DATA_BLOCK "ALLARMI_MP270"
AUTHOR : LD
FAMILY : DESTACK
NAME : ALLARMI
VERSION : 0.1


  STRUCT
   Allar_9 : BOOL ;	//Magnetotermici 24 Volt drive
   Allar_10 : BOOL ;	//Magnetotermico alimentazione uscite plc
   Allar_11 : BOOL ;	//Magnetotermico alimentazione ingressi plc
   Allar_12 : BOOL ;	//Magnetotermico traslazione tavola 1
   Allar_13 : BOOL ;	//Magnetotermico traslazione tavola 2
   Allar_14 : BOOL ;	//Magnetotermico pompa tavola 1
   Allar_15 : BOOL ;	//Magnetotermico pompa tavola 2
   Allar_16 : BOOL ;	//Magnetotermico regolazione altezza sfogliatore
   Allar_1 : BOOL ;	//Emergenze da ripristinare
   Allar_2 : BOOL ;	//Emergenza pannello di comando
   Allar_3 : BOOL ;	//Emergenza sfogliatore lato operatore
   Allar_4 : BOOL ;	//Emergenza porta sfogliatore lato opposto operatore
   Allar_5 : BOOL ;	//Emergenza porta lato operatore
   Allar_6 : BOOL ;	//Emergenza porta lato opposto operatore
   Allar_7 : BOOL ;	//Porta aperta lato operatore
   Allar_8 : BOOL ;	//Porta aperta lato opposto operatore
   Allar_25 : BOOL ;	//Magnetotermico ventilatore armadio
   Allar_26 : BOOL ;	//Magnetotermico generale ausiliari
   Allar_27 : BOOL ;	//Antischiacciamento tavola 1 sx
   Allar_28 : BOOL ;	//Antischiacciamento tavola 2 dx
   Allar_29 : BOOL ;	//Anticollisione tavola 1 sx
   Allar_30 : BOOL ;	//Anticollisione tavola 2 dx
   Allar_31 : BOOL ;	//Oltrecorsa salita tavola
   Allar_32 : BOOL ;	//Barriera di sicurezza dx lato opposto operatore
   Allar_17 : BOOL ;	//Magnetotermico regolazione altezza centratore
   Allar_18 : BOOL ;	//Magnetotermico traslazione centratore
   Allar_19 : BOOL ;	//Magnetotermico regolazione posteriore sx centratore
   Allar_20 : BOOL ;	//Magnetotermico regolazione posteriore dx centratore
   Allar_21 : BOOL ;	//Magnetotermico regolazione anteriore sx centratore
   Allar_22 : BOOL ;	//Magnetotermico regolazione anteriore dx centratore
   Allar_23 : BOOL ;	//Magnetotermico regolazione laterale dx centratore
   Allar_24 : BOOL ;	//Magnetotermico regolazione laterale sx centratore
   Allar_41 : BOOL ;	//Sicurezze antischiacc.e anticollisione escluse
   Allar_42 : BOOL ;	//Disfunzione micro P.E. su centratore
   Allar_43 : BOOL ;	//Riserva
   Allar_44 : BOOL ;	//Selezione cambio produzione manuale inserito
   Allar_45 : BOOL ;	//Richiesta apertura isola 1
   Allar_46 : BOOL ;	//Anomalia drive centratore Posteriore DX
   Allar_47 : BOOL ;	//Anomalia drive centratore Laerale DX
   Allar_48 : BOOL ;	//Anomalia drive centratore Laerale SX
   Allar_33 : BOOL ;	//Allarme su AP&T
   Allar_34 : BOOL ;	//Matricola non caricata da AP&T
   Allar_35 : BOOL ;	//Magneti non in posizione
   Allar_36 : BOOL ;	//Portare AP&T in posizione di inizio ciclo
   Allar_37 : BOOL ;	//Anomalia drive centratore Anteriore DX
   Allar_38 : BOOL ;	//Anomalia drive centratore Anteriore SX
   Allar_39 : BOOL ;	//Anomalia drive centratore Posteriore DX
   Allar_40 : BOOL ;	//Posizionare ABB in cambio produzione
   Allar_57 : BOOL ;	//Fine pacco tranciati su tavola
   Allar_58 : BOOL ;	//Riserva
   Allar_59 : BOOL ;	//Pressa non al P.M.S.
   Allar_60 : BOOL ;	//Spina start pressa non inserita
   Allar_61 : BOOL ;	//FC TAVOLA 1 lato disimpilamento
   Allar_62 : BOOL ;	//FC TAVOLA 2 lato disimpilamento
   Allar_63 : BOOL ;	//Allarme da robot perdita pezzo
   Allar_64 : BOOL ;	//Allarme riparo aperto isola 1
   Allar_49 : BOOL ;	//Lamiera nello stampo
   Allar_50 : BOOL ;	//Lamiera su centraggio in ciclo di cambio produzione
   Allar_51 : BOOL ;	//Pressa non pronta per auto
   Allar_52 : BOOL ;	//Doppio foglio
   Allar_53 : BOOL ;	//Robot non pronto per auto
   Allar_54 : BOOL ;	//Assenza foglio su stazione di centraggio
   Allar_55 : BOOL ;	//Braccio ABB non in posizione di produzione
   Allar_56 : BOOL ;	//Attesa pezzo prelevato dallo stampo (robot isola1)
   Allar_73 : BOOL ;	//Ciclo cambio matricola in corso
   Allar_74 : BOOL ;	//Ciclo cambio pacco in corso
   Allar_75 : BOOL ;	//Sicurezza magneti sfogliatore
   Allar_76 : BOOL ;	//Pacco non arrivato in posizione di sfogliatura
   Allar_77 : BOOL ;	//Tavola 1 non in finecorsa lato caricamento (indietro
   Allar_78 : BOOL ;	//Tavola 2 non in finecorsa lato caricamento (indietro
   Allar_79 : BOOL ;	//Magneti sfogliatori non rientrati
   Allar_80 : BOOL ;	//Riserva
   Allar_65 : BOOL ;	//Barriera di sicurezza sx lato operatore
   Allar_66 : BOOL ;	//cancelletti tavola 1
   Allar_67 : BOOL ;	//cancelletti tavola 2x
   Allar_68 : BOOL ;	//Unita' di centraggio sbloccata
   Allar_69 : BOOL ;	//Cambio matricola quota non raggiunta
   Allar_70 : BOOL ;	//Batteria plc scarica
   Allar_71 : BOOL ;	//Tavola 1 non abbassata
   Allar_72 : BOOL ;	//Tavola 2 non abbassata
   Allar_89 : BOOL ;	//Contemporaneita' fc  traslazione tavola 1
   Allar_90 : BOOL ;	//Contemporaneita' fc  traslazione tavola 2
   Allar_91 : BOOL ;	//Contemporaneita' fc regolazione altezza sfogliatore
   Allar_92 : BOOL ;	//Contemporaneita' fc  regolazione altezza centraggio
   Allar_93 : BOOL ;	//Contemporaneita' fc  traslazione centratore
   Allar_94 : BOOL ;	//Contemporaneita' fc  regolazione centraggio post.SX
   Allar_95 : BOOL ;	//Contemporaneita' fc  regolazione centraggio post.DX
   Allar_96 : BOOL ;	//Contemporaneita' fc  regolazione centraggio ant.
   Allar_81 : BOOL ;	//Muting inserito tavola 1
   Allar_82 : BOOL ;	//Muting inserito tavola 2
   Allar_83 : BOOL ;	//Comandi disinseriti
   Allar_84 : BOOL ;	//Braccio ABB in posizione di prelievo
   Allar_85 : BOOL ;	//Anomalia vuoto su centratore
   Allar_86 : BOOL ;	//Anomalia vuoto su sfogliatore
   Allar_87 : BOOL ;	//Quota tavola non raggiunta
   Allar_88 : BOOL ;	//Selettore programmazione inserito
   Allar_105 : BOOL ;	//Anomalia fc  tavola 1 avanti lato dispilamento
   Allar_106 : BOOL ;	//Anomalia fc  tavola 1 indietro lato carico
   Allar_107 : BOOL ;	//Anomalia fc  tavola 2 avanti lato dispilamento
   Allar_108 : BOOL ;	//Anomalia fc  tavola 2 indietro lato carico
   Allar_109 : BOOL ;	//Zero assi centratore da eseguire
   Allar_110 : BOOL ;	//Inserire nuovo codice matricola
   Allar_111 : BOOL ;	//Sostituire tooling e premere C.P. start
   Allar_112 : BOOL ;	//Tavola di centraggio non bloccata
   Allar_97 : BOOL ;	//Selezione cambio produzione in automatico
   Allar_98 : BOOL ;	//Contemporaneita' fc  centratura laterale dx
   Allar_99 : BOOL ;	//Contemporaneita' fc centratura laterale sx
   Allar_100 : BOOL ;	//Time out centraggi longitudinali fuori
   Allar_101 : BOOL ;	//Time out centraggi laterale fuori
   Allar_102 : BOOL ;	//Contemporaneita' fc blocc/sblocc centratore
   Allar_103 : BOOL ;	//Contemporaneita' fc  sollevamento tavola 1
   Allar_104 : BOOL ;	//Contemporaneita' fc  sollevamento tavola 2
   Allar_121 : BOOL ;	//Assenza pedana materiale su tavola zona sfogliatura
   Allar_122 : BOOL ;	//Fotocellula 45B1 H200 guasta o disallineata
   Allar_123 : BOOL ;	//Fotocellula 45B3 H120 guasta o disallineata
   Allar_124 : BOOL ;	//Salire con la tavola in manuale
   Allar_125 : BOOL ;	//Anomalia dispositivo Klaska (cavo interrotto)
   Allar_126 : BOOL ;	//Time out Unita' di centraggio bloccata
   Allar_127 : BOOL ;	//Time out Unita' di centraggio sbloccata
   Allar_128 : BOOL ;	//Magnetotermico trasformatore brushless centratori (12QF2)
   Allar_113 : BOOL ;	//Motori ABB non inseriti
   Allar_114 : BOOL ;	//Cambio pacco prenotato
   Allar_115 : BOOL ;
   Allar_116 : BOOL ;	//Tavole 1 e 2  in muting
   Allar_117 : BOOL ;	//Klascka non rileva sequenza 2Fogli, 1Foglio, 0Fogli
   Allar_118 : BOOL ;	//Klascka non rileva 2 fogli nel prelievo
   Allar_119 : BOOL ;	//Klascka rileva 0 fogli nel ciclo di carico
   Allar_120 : BOOL ;	//Braccio ABB non in posizione di prelievo
   Allar_137 : BOOL ;	//Time out salita regolazione altezza centratore
   Allar_138 : BOOL ;	//Time out discesa regolazione altezza centratore
   Allar_139 : BOOL ;	//Time out centratore verso pressa
   Allar_140 : BOOL ;	//Time out centratore verso sfogliatore
   Allar_141 : BOOL ;	//Time out indietro magnete 1
   Allar_142 : BOOL ;	//Time out avanti magnete 1
   Allar_143 : BOOL ;	//Time out indietro magnete 2
   Allar_144 : BOOL ;	//Time out avanti magnete 2
   Allar_129 : BOOL ;	//Contemporaneita' fc magnete 1
   Allar_130 : BOOL ;	//Contemporaneita' fc magnete 2
   Allar_131 : BOOL ;	//Contemporaneita' fc magnete 3
   Allar_132 : BOOL ;	//Contemporaneita' fc magnete 4
   Allar_133 : BOOL ;	//Contemporaneita' fc magnete 5
   Allar_134 : BOOL ;	//Contemporaneita' fc magnete 6
   Allar_135 : BOOL ;	//Contemporaneita' fc magnete laterale sx
   Allar_136 : BOOL ;	//Contemporaneita' fc magnete laterale dx
   Allar_153 : BOOL ;	//Time out indietro magnete laterale sx
   Allar_154 : BOOL ;	//Time out avanti magnete laterale sx
   Allar_155 : BOOL ;	//Time out indietro magnete laterale dx
   Allar_156 : BOOL ;	//Time out avanti magnete laterale dx
   Allar_157 : BOOL ;	//Time out chiusura braccio magnete laterale sx
   Allar_158 : BOOL ;	//Time out apertura braccio magnete laterale sx
   Allar_159 : BOOL ;	//Time out chiusura braccio magnete laterale dx
   Allar_160 : BOOL ;	//Time out apertura braccio magnete laterale dx
   Allar_145 : BOOL ;	//Time out indietro magnete 3
   Allar_146 : BOOL ;	//Time out avanti magnete 3
   Allar_147 : BOOL ;	//Time out indietro magnete 4
   Allar_148 : BOOL ;	//Time out avanti magnete 4
   Allar_149 : BOOL ;	//Time out indietro magnete 5
   Allar_150 : BOOL ;	//Time out avanti magnete 5
   Allar_151 : BOOL ;	//Time out indietro magnete 6
   Allar_152 : BOOL ;	//Time out avanti magnete 6
   Allar_169 : BOOL ;	//Porta aperta sfogliatore lato dx
   Allar_170 : BOOL ;	//Porta aperta sfogliatore lato sx
   Allar_171 : BOOL ;	//Extracorsa avanti tavola 1
   Allar_172 : BOOL ;	//Extracorsa avanti tavola 2
   Allar_173 : BOOL ;	//Extracorsa indietro tavola 1
   Allar_174 : BOOL ;	//Extracorsa indietro tavola 2
   Allar_175 : BOOL ;	//Emergenza ABB
   Allar_176 : BOOL ;	//Extracorsa incremento pacco (fc su braccio ABB)
   Allar_161 : BOOL ;	//Carro non in posizione di riposo
   Allar_162 : BOOL ;	//Periferia decentrata Destacker in errore
   Allar_163 : BOOL ;	//Periferia decentrata AP&T in errore
   Allar_164 : BOOL ;	//Ciclo AP&T non coerente
   Allar_165 : BOOL ;	//E60.4 Magnete Ausiliario 1 Tavola 1 non rientrato
   Allar_166 : BOOL ;	//E60.6 Magnete Ausiliario 2 Tavola 1 non rientrato
   Allar_167 : BOOL ;	//E70.4 Magnete Ausiliario 1 Tavola 2 non rientrato
   Allar_168 : BOOL ;	//E70.6 Magnete Ausiliario 2 Tavola 2 non rientrato
   Allar_185 : BOOL ;	//Attenzione!  dovresti aprire i centraggi
   Allar_186 : BOOL ;	//Emergenza linea Comau da ripristinare
   Allar_187 : BOOL ;	//Ripristinare sensore presenza su braccio ABB
   Allar_188 : BOOL ;	//Mancanza improvvisa consenso ingr.pressa
   Allar_189 : BOOL ;	//ABB non in start auto  (ciclo in corso)
   Allar_190 : BOOL ;	//Posizionare i gruppi a riposo per cambio tooling
   Allar_191 : BOOL ;	//Retrofitting pulsanti EM non premuti per comau
   Allar_192 : BOOL ;	//Retrofitting Ripari chiusi per ABB
   Allar_177 : BOOL ;	//Tavola 1 piena in uscita
   Allar_178 : BOOL ;	//Tavola 2 piena in uscita
   Allar_179 : BOOL ;	//Retrofitting rele' ciclo automatico destacker
   Allar_180 : BOOL ;	//Retrofitting rele' ripari/barriere destacker
   Allar_181 : BOOL ;	//Retrofitting rele' start pressa (per comau)
   Allar_182 : BOOL ;	//Retrofitting Rele' emergenza Destaker
   Allar_183 : BOOL ;	//Retrofitting anticollisione/antischiacciamento tavole
   Allar_184 : BOOL ;	//Retrofitting override barriere
   word_3042 : BOOL ;
   word_3043 : BOOL ;
   word_3044 : BOOL ;
   word_3045 : BOOL ;
   word_3046 : BOOL ;
   word_3047 : BOOL ;
   word_3048 : BOOL ;
   word_3049 : BOOL ;
   word_3050 : BOOL ;
   word_3051 : BOOL ;
   word_3052 : BOOL ;
   word_3053 : BOOL ;
   word_3054 : BOOL ;
   word_3055 : BOOL ;
   word_3056 : BOOL ;
   word_3057 : BOOL ;
   Allar_217 : BOOL ;	//Porta 2: non abilitata alla marcia
   Allar_218 : BOOL ;	//Porta 2: time-out discesa porta o non chiusa
   Allar_219 : BOOL ;	//Porta 2: time-out salita porta o non aperta
   Allar_220 : BOOL ;	//Porta 2: carro non in posizione per ciclo porta
   Allar_221 : BOOL ;	//Porta 2: livello di traslazione carro 2 troppo alto
   word_3063 : BOOL ;
   word_3064 : BOOL ;
   word_3065 : BOOL ;
   Allar_209 : BOOL ;	//Porta 1: non abilitata alla marcia
   Allar_210 : BOOL ;	//Porta 1: time-out discesa porta o non chiusa
   Allar_211 : BOOL ;	//Porta 1: time-out salita porta o non aperta
   Allar_212 : BOOL ;	//Porta 1: carro non in posizione per ciclo porta
   Allar_213 : BOOL ;	//Porta 1: livello di traslazione carro 1 troppo alto
   word_30635 : BOOL ;
   word_30636 : BOOL ;
   word_30637 : BOOL ;
   word_30638 : BOOL ;
   word_30639 : BOOL ;
   word_306310 : BOOL ;
   word_306311 : BOOL ;
   word_306312 : BOOL ;
   word_306313 : BOOL ;
   word_306314 : BOOL ;
   word_306315 : BOOL ;
   Allar_225 : BOOL ;	//Porta 1 e 2: magnetotermico linea alimentazione porte 1 e 2
   word_3063152 : BOOL ;
   word_3063153 : BOOL ;
   word_30631531 : BOOL ;
   word_30631532 : BOOL ;
   word_30631533 : BOOL ;
   word_30631534 : BOOL ;
   word_30631535 : BOOL ;
   Da_APT_allarme_1 : BOOL ;	//SF1 - A: Pezzo caduto in pinza I @1D%5.1f@
   Da_APT_allarme_2 : BOOL ;	//SF1 - M: Non riceve il pezzo nella pinza I@1D%5.1f@
   Da_APT_allarme_3 : BOOL ;	//SF1 - W: Intermittenza vuoto troppo elevata nell'unità di presa I@1D%5.1f@
   Da_APT_allarme_4 : BOOL ;	//SF1 - A: Errore unità di presa protezione vuoto I@1D%5.1f@
   Da_APT_allarme_5 : BOOL ;	//SF1 - W: Errore unità di presa aperta I@1D%5.1f@
   Da_APT_allarme_6 : BOOL ;	//SF1 - A: Comando stop salto sequenza
   Da_APT_allarme_7 : BOOL ;	//SF1 - M: Avvio forzato
   Da_APT_allarme_8 : BOOL ;	//SF1 - A: L'asse X1_A1 ha perduto la regolazione
   Da_APT_allarme_9 : BOOL ;	//SF1 - A: Doppio Foglio UC70
   Da_APT_allarme_10 : BOOL ;	//SF1 – A: Errore di calibrazione controllo Doppio Foglio UC70
   Da_APT_allarme_11 : BOOL ;	//SF1 - M: Assi non innestati
   Da_APT_allarme_12 : BOOL ;	//SF1 - A: Perdita innesto assi
   Da_APT_allarme_13 : BOOL ;	//RISERVA
   Da_APT_allarme_14 : BOOL ;	//SF1 - A: Posizione o salto fuori limiti - fase - Check MP177
   Da_APT_allarme_15 : BOOL ;	//SF1 - A: Errore coordinate parametri di impilamento 1
   Da_APT_allarme_16 : BOOL ;	//SF1 - A: Timeout per richiesta apertura protezione
   Da_APT_allarme_17 : BOOL ;	//SF1 - A: Errore avanzamento asse
   Da_APT_allarme_18 : BOOL ;	//SF1 - A: Errore calibrazione asse
   Da_APT_allarme_19 : BOOL ;	//SF1 - M: Movimento in Z- non possibile per intervento Klaschka
   Da_APT_allarme_20 : BOOL ;	//SF1 - A: Timeout per misurazione/calibrazione nel controllo Doppio Foglio
   Da_APT_allarme_21 : BOOL ;	//SF1 - M: Quantità impostata raggiunta - contatore 1
   Da_APT_allarme_22 : BOOL ;	//SF1 - M: Quantità impostata raggiunta - contatore 2
   Da_APT_allarme_23 : BOOL ;	//SF1 - A: Stop da Linea
   Da_APT_allarme_24 : BOOL ;	//RISERVA
   Da_APT_allarme_25 : BOOL ;	//SF1 - A: Ripari aperti
   Da_APT_allarme_26 : BOOL ;	//A1624 – M:Intervento disgiuntore, controllare alimentazione a unità QF860
   Da_APT_allarme_27 : BOOL ;	//SF1  A: Nessun dettaglio trovato sulla navetta di alimentazione
   Da_APT_allarme_28 : BOOL ;	//SF1 - A: Parte imprevista su navetta
   Da_APT_allarme_29 : BOOL ;	//SF1 - M: Ripari aperti o non ripristinati
   Da_APT_allarme_30 : BOOL ;	//RISERVA
   Da_APT_allarme_31 : BOOL ;	//RISERVA
   Da_APT_allarme_32 : BOOL ;	//RISERVA
   Da_APT_allarme_33 : BOOL ;	//RISERVA
   Da_APT_allarme_34 : BOOL ;	//SF1 - M: Timeout cambio ricetta
   Da_APT_allarme_35 : BOOL ;	//A1624 - M: Trasportatore pieno
   Da_APT_allarme_36 : BOOL ;	//A1624 - A: Interruttore del nastro trasportatore scattato
   Da_APT_allarme_37 : BOOL ;	//A1624 - M:Arresto di emergenza interno attivato
   Da_APT_allarme_38 : BOOL ;	//SF1 - M: Pallet 1 completo - Cambiare pallet
   Da_APT_allarme_39 : BOOL ;	//SF1 - M: Pallet 2 completo - Cambiare pallet
   Da_APT_allarme_40 : BOOL ;	//SF1 - A: Arresto da controllo estrattore
   Da_APT_allarme_41 : BOOL ;	//SF1 - M: Nessuna parte in posizione su navetta
   Da_APT_allarme_42 : BOOL ;	//SF1 - A: Parte imprevista su navetta
   Da_APT_allarme_43 : BOOL ;	//SF1 - A: L'asse X1_A1 ha perduto la regolazione
   Da_APT_allarme_44 : BOOL ;	//SF1 - A: L'asse Y_A1 ha perduto la regolazione
   Da_APT_allarme_45 : BOOL ;	//SF1 - A: L'asse Z_A1 ha perduto la regolazione
   Da_APT_allarme_46 : BOOL ;	//SF1 - A: L'asse A_A1 ha perduto la regolazione
   Da_APT_allarme_47 : BOOL ;	//SF1 - A: Pressa non in posizione superiore
   Da_APT_allarme_48 : BOOL ;	//SF1 - A: Basculamento non alto
   Da_APT_allarme_49 : BOOL ;	//A1624 - W: Guasto nella navetta del motore dell'attacco laterale
   Da_APT_allarme_50 : BOOL ;	//A1624 - A: Nessuna connessione al PLC A500 di sicurezza
   Da_APT_allarme_51 : BOOL ;	//RISERVA
   Da_APT_allarme_52 : BOOL ;	//SF1 - A: Errore di sicurezza integrata. Ripristinare la SI o riavviare
   Da_APT_allarme_53 : BOOL ;	//SF1 - A: Parte rilasciata, unità di presa troppo calda
   Da_APT_allarme_54 : BOOL ;	//SF1 - A: Timeout per unità di presa calda, azionare per sfridi
   Da_APT_allarme_55 : BOOL ;	//SF1 - M:Timeout per unità di presa calda, lasciare parte nell'utensile
   Da_APT_allarme_56 : BOOL ;	//SF1 - W: Protezione da surriscaldamento per pinza bloccata
   Da_APT_allarme_57 : BOOL ;	//SF1 A: il valore limite pressa non rientra nell'intervallo programmato
   Da_APT_allarme_58 : BOOL ;	//A1624 - g_i_ERROR[58]
   Da_APT_allarme_59 : BOOL ;	//A1624 - g_i_ERROR[59]
   Da_APT_allarme_60 : BOOL ;	//A1624 - g_i_ERROR[60]
   Da_APT_allarme_61 : BOOL ;	//A1624 - g_i_ERROR[61]
   Da_APT_allarme_62 : BOOL ;	//RISERVA
   Da_APT_allarme_63 : BOOL ;	//RISERVA
   Da_APT_allarme_64 : BOOL ;	//RISERVA
   Da_APT_allarme_65 : BOOL ;	//RISERVA
   Da_APT_allarme_66 : BOOL ;	//RISERVA
   Da_APT_allarme_67 : BOOL ;	//RISERVA
   Da_APT_allarme_68 : BOOL ;	//RISERVA
   Da_APT_allarme_69 : BOOL ;	//RISERVA
   Da_APT_allarme_70 : BOOL ;	//A1624 - M: Nessuna comunicazione - unità linea
   Da_APT_allarme_71 : BOOL ;	//A1624 - W: Tensione batteria bassa K600
   Da_APT_allarme_72 : BOOL ;	//A1624 - A: Errore dell'unità servoalimentatore TA700 - UH1
   Da_APT_allarme_73 : BOOL ;	//A1624 - A: Malfunzionamento nel contattore principale QA700 -UH1
   Da_APT_allarme_74 : BOOL ;	//RISERVA
   Da_APT_allarme_75 : BOOL ;	//A1624 - M: Modalità test attiva
   Da_APT_allarme_76 : BOOL ;	//SF1 - A: Arresto di emergenza interno MP177. K75-1
   Da_APT_allarme_77 : BOOL ;	//A1624 - A: Arresto di emergenza esterno
   Da_APT_allarme_78 : BOOL ;	//A1624 - A: Feedback safe 24V non OK - S
   Da_APT_allarme_79 : BOOL ;	//SF1 - A: Sovraccarico asse X1_A1
   Da_APT_allarme_80 : BOOL ;	//SF1 - A: Sovraccarico asse Z_A1
   Da_APT_allarme_81 : BOOL ;	//SF1 - A: Sovraccarico asse Y_A1
   Da_APT_allarme_82 : BOOL ;	//SF1 - A: Sovraccarico asse A_A1
   Da_APT_allarme_83 : BOOL ;	//A1624 - M: Livello dell'olio dell'unità di lubrificazione basso
   Da_APT_allarme_84 : BOOL ;	//A1624 - g_i_ERROR[84]
   Da_APT_allarme_85 : BOOL ;	//A1624 - g_i_ERROR[85]
   Da_APT_allarme_86 : BOOL ;	//A1624 - g_i_ERROR[86]
   Da_APT_allarme_87 : BOOL ;	//A1624 - g_i_ERROR[87]
   Da_APT_allarme_88 : BOOL ;	//RISERVA
   Da_APT_allarme_89 : BOOL ;	// - M: Unità di lubrificazione non accesa
   Da_APT_allarme_90 : BOOL ;	//A1624 - A: Il cilindro raccoglitore HSD non riceve il vuoto
   Da_APT_allarme_91 : BOOL ;	//A1624 - M: Raspa non in pos. interna HSD
   Da_APT_allarme_92 : BOOL ;	//A1624 - A: Telaio di sicurezza HSD scattato
   Da_APT_allarme_93 : BOOL ;	//A1624 - A: Deposito HSD non in posizione
   Da_APT_allarme_94 : BOOL ;	//SF1 - A: Assi esterni ai limiti dell'accoppiamento automatico
   Da_APT_allarme_95 : BOOL ;	//SF1 - M: Parametri di manovra modificati - Riavviare controllo sistema
   Da_APT_allarme_96 : BOOL ;	//SF1 - A: Errore di download dei parametri
   Da_APT_allarme_97 : BOOL ;	//BF - M: Protezioni aperte o non ripristinate - Deposito 1
   Da_APT_allarme_98 : BOOL ;	//BF - M: Protezioni aperte o non ripristinate - Deposito 2
   Da_APT_allarme_99 : BOOL ;	//A1624 - M: Ripristino della sicurezza integrata
   Da_APT_allarme_100 : BOOL ;	//A1624 - M: Fusibile F1 scattato - Armadio UH1
   Da_APT_allarme_101 : BOOL ;	//A1624 - M: Fusibile F5 scattato - Armadio UH1
   Da_APT_allarme_102 : BOOL ;	//A1624 - M: Fusibile F6 scattato - Armadio UH1
   Da_APT_allarme_103 : BOOL ;	//A1624 - M: Fusibile F860 scattato - Armadio UH1
   Da_APT_allarme_104 : BOOL ;	//A1624 - W: Unità di raffreddamento non funzionante - Armadio UH1
   Da_APT_allarme_105 : BOOL ;	//A1624 - A: Profisafe I/O richiede conferma
   Da_APT_allarme_106 : BOOL ;	//A1624 - A: Feedback per arresto di emergenza non OK I17.0
   Da_APT_allarme_107 : BOOL ;	//A1624 - A: Arresto di emergenza interno ARxxx
   Da_APT_allarme_108 : BOOL ;	//A1624 - A: Arresto di emergenza interno ARxxx
   Da_APT_allarme_109 : BOOL ;	//A1624 - A: Arresto di emergenza interno MP177 COIL
   Da_APT_allarme_110 : BOOL ;	//A1624 - M: Fusibile F1 scattato - Armadio UH2
   Da_APT_allarme_111 : BOOL ;	//A1624 - M: Fusibile F5 scattato - Armadio UH2
   Da_APT_allarme_112 : BOOL ;	//A1624 - M: Fusibile F6 scattato - Armadio UH2
   Da_APT_allarme_113 : BOOL ;	//A1624 - M: Fusibile F860 scattato - Armadio UH2
   Da_APT_allarme_114 : BOOL ;	//A1624 - W: Unità di raffreddamento non operativo - Cabinet UH2
   Da_APT_allarme_115 : BOOL ;	//SF1 - A: Errore dell'asse X1_A1
   Da_APT_allarme_116 : BOOL ;	//SF1 - A: Errore dell'asse Z_A1
   Da_APT_allarme_117 : BOOL ;	//SF1 - A: Errore dell'asse Y_A1
   Da_APT_allarme_118 : BOOL ;	//SF1 - A: Errore dell'asse A_A1
   Da_APT_allarme_119 : BOOL ;	//RISERVA
   Da_APT_allarme_120 : BOOL ;	//SF1 - A: Arresto dalla macchina esterna - PS1 (Pressa)
   Da_APT_allarme_121 : BOOL ;	//SF1 - A: Arresto dalla macchina esterna - PS2 (Comau robot)
   Da_APT_allarme_122 : BOOL ;	//SF1 - A: Arresto dalla macchina esterna - PS3
   Da_APT_allarme_123 : BOOL ;	//SF1 - A: Arresto dalla macchina esterna - PS4
   Da_APT_allarme_124 : BOOL ;	//SF1 - A: Perdita pezzo - Sfogliatore - I10.4
   Da_APT_allarme_125 : BOOL ;	//SF1 - A: Perdita pezzo - Sfogliatore - I10.5
   Da_APT_allarme_126 : BOOL ;	//SF1 - A: Perdita pezzo - Centraggio - I10.6
   Da_APT_allarme_127 : BOOL ;	//SF1 - A: Perdita pezzo - Centraggio - I10.7
   Da_APT_allarme_128 : BOOL ;	//SF1 - M: Pezzo non prelevato - Sfogliatore - I10.4
   Da_APT_allarme_129 : BOOL ;	//SF1 - M: Pezzo non prelevato - Sfogliatore - I10.5
   Da_APT_allarme_130 : BOOL ;	//SF1 - M: Pezzo non prelevato - Centraggio - I10.6
   Da_APT_allarme_131 : BOOL ;	//SF1 - M: Pezzo non prelevato - Centraggio - I10.7
   Da_APT_allarme_132 : BOOL ;	//SF1 - W: Amolalia vuoto - Sfogliatore - I10.4
   Da_APT_allarme_133 : BOOL ;	//SF1 - W: Amolalia vuoto - Sfogliatore - I10.5
   Da_APT_allarme_134 : BOOL ;	//SF1 - W: Amolalia vuoto - Centraggio - I10.6
   Da_APT_allarme_135 : BOOL ;	//SF1 - W: Amolalia vuoto - Centraggio - I10.7
   Da_APT_allarme_136 : BOOL ;	//SF1 - A: Anomalia vacuostato - Sfogliatore - I10.4
   Da_APT_allarme_137 : BOOL ;	//SF1 - A: Anomalia vacuostato - Sfogliatore - I10.5
   Da_APT_allarme_138 : BOOL ;	//SF1 - A: Anomalia vacuostato - Centraggio - I10.6
   Da_APT_allarme_139 : BOOL ;	//SF1 - A: Anomalia vacuostato - Centraggio - I10.7
   Da_APT_allarme_140 : BOOL ;	//SF1 - M: Richiesta Svuotamento Linea
   Da_APT_allarme_141 : BOOL ;	//SF1 - A: Spare application Nr 10
   Da_APT_allarme_142 : BOOL ;	//SF1 - A: Spare application Nr 9
   Da_APT_allarme_143 : BOOL ;	//SF1 - A: Spare application Nr 8
   Da_APT_allarme_144 : BOOL ;	//SF1 - A: Spare application Nr 7
   Da_APT_allarme_145 : BOOL ;
   Da_APT_allarme_146 : BOOL ;
   Da_APT_allarme_147 : BOOL ;
   Da_APT_allarme_148 : BOOL ;
   Da_APT_allarme_149 : BOOL ;
   Da_APT_allarme_150 : BOOL ;
   Da_APT_allarme_151 : BOOL ;
   Da_APT_allarme_152 : BOOL ;
   Da_APT_allarme_153 : BOOL ;
   Da_APT_allarme_154 : BOOL ;
   Da_APT_allarme_155 : BOOL ;
   Da_APT_allarme_156 : BOOL ;
   Da_APT_allarme_157 : BOOL ;
   Da_APT_allarme_158 : BOOL ;
   Da_APT_allarme_159 : BOOL ;
   Da_APT_allarme_160 : BOOL ;
  END_STRUCT ;
BEGIN
   Allar_9 := FALSE;
   Allar_10 := FALSE;
   Allar_11 := FALSE;
   Allar_12 := FALSE;
   Allar_13 := FALSE;
   Allar_14 := FALSE;
   Allar_15 := FALSE;
   Allar_16 := FALSE;
   Allar_1 := FALSE;
   Allar_2 := FALSE;
   Allar_3 := FALSE;
   Allar_4 := FALSE;
   Allar_5 := FALSE;
   Allar_6 := FALSE;
   Allar_7 := FALSE;
   Allar_8 := FALSE;
   Allar_25 := FALSE;
   Allar_26 := FALSE;
   Allar_27 := FALSE;
   Allar_28 := FALSE;
   Allar_29 := FALSE;
   Allar_30 := FALSE;
   Allar_31 := FALSE;
   Allar_32 := FALSE;
   Allar_17 := FALSE;
   Allar_18 := FALSE;
   Allar_19 := FALSE;
   Allar_20 := FALSE;
   Allar_21 := FALSE;
   Allar_22 := FALSE;
   Allar_23 := FALSE;
   Allar_24 := FALSE;
   Allar_41 := FALSE;
   Allar_42 := FALSE;
   Allar_43 := FALSE;
   Allar_44 := FALSE;
   Allar_45 := FALSE;
   Allar_46 := FALSE;
   Allar_47 := FALSE;
   Allar_48 := FALSE;
   Allar_33 := FALSE;
   Allar_34 := FALSE;
   Allar_35 := FALSE;
   Allar_36 := FALSE;
   Allar_37 := FALSE;
   Allar_38 := FALSE;
   Allar_39 := FALSE;
   Allar_40 := FALSE;
   Allar_57 := FALSE;
   Allar_58 := FALSE;
   Allar_59 := FALSE;
   Allar_60 := FALSE;
   Allar_61 := FALSE;
   Allar_62 := FALSE;
   Allar_63 := FALSE;
   Allar_64 := FALSE;
   Allar_49 := FALSE;
   Allar_50 := FALSE;
   Allar_51 := TRUE;
   Allar_52 := FALSE;
   Allar_53 := FALSE;
   Allar_54 := FALSE;
   Allar_55 := FALSE;
   Allar_56 := FALSE;
   Allar_73 := FALSE;
   Allar_74 := FALSE;
   Allar_75 := FALSE;
   Allar_76 := FALSE;
   Allar_77 := FALSE;
   Allar_78 := FALSE;
   Allar_79 := FALSE;
   Allar_80 := FALSE;
   Allar_65 := FALSE;
   Allar_66 := FALSE;
   Allar_67 := FALSE;
   Allar_68 := FALSE;
   Allar_69 := FALSE;
   Allar_70 := FALSE;
   Allar_71 := FALSE;
   Allar_72 := FALSE;
   Allar_89 := FALSE;
   Allar_90 := FALSE;
   Allar_91 := FALSE;
   Allar_92 := FALSE;
   Allar_93 := FALSE;
   Allar_94 := FALSE;
   Allar_95 := FALSE;
   Allar_96 := FALSE;
   Allar_81 := FALSE;
   Allar_82 := FALSE;
   Allar_83 := FALSE;
   Allar_84 := FALSE;
   Allar_85 := FALSE;
   Allar_86 := FALSE;
   Allar_87 := FALSE;
   Allar_88 := FALSE;
   Allar_105 := FALSE;
   Allar_106 := FALSE;
   Allar_107 := FALSE;
   Allar_108 := FALSE;
   Allar_109 := FALSE;
   Allar_110 := FALSE;
   Allar_111 := FALSE;
   Allar_112 := FALSE;
   Allar_97 := FALSE;
   Allar_98 := FALSE;
   Allar_99 := FALSE;
   Allar_100 := FALSE;
   Allar_101 := FALSE;
   Allar_102 := FALSE;
   Allar_103 := FALSE;
   Allar_104 := FALSE;
   Allar_121 := FALSE;
   Allar_122 := FALSE;
   Allar_123 := FALSE;
   Allar_124 := FALSE;
   Allar_125 := FALSE;
   Allar_126 := FALSE;
   Allar_127 := FALSE;
   Allar_128 := FALSE;
   Allar_113 := FALSE;
   Allar_114 := FALSE;
   Allar_115 := FALSE;
   Allar_116 := FALSE;
   Allar_117 := FALSE;
   Allar_118 := FALSE;
   Allar_119 := FALSE;
   Allar_120 := FALSE;
   Allar_137 := FALSE;
   Allar_138 := FALSE;
   Allar_139 := FALSE;
   Allar_140 := FALSE;
   Allar_141 := FALSE;
   Allar_142 := FALSE;
   Allar_143 := FALSE;
   Allar_144 := FALSE;
   Allar_129 := FALSE;
   Allar_130 := FALSE;
   Allar_131 := FALSE;
   Allar_132 := FALSE;
   Allar_133 := FALSE;
   Allar_134 := FALSE;
   Allar_135 := FALSE;
   Allar_136 := FALSE;
   Allar_153 := FALSE;
   Allar_154 := FALSE;
   Allar_155 := FALSE;
   Allar_156 := FALSE;
   Allar_157 := FALSE;
   Allar_158 := FALSE;
   Allar_159 := FALSE;
   Allar_160 := FALSE;
   Allar_145 := FALSE;
   Allar_146 := FALSE;
   Allar_147 := FALSE;
   Allar_148 := FALSE;
   Allar_149 := FALSE;
   Allar_150 := FALSE;
   Allar_151 := FALSE;
   Allar_152 := FALSE;
   Allar_169 := FALSE;
   Allar_170 := FALSE;
   Allar_171 := FALSE;
   Allar_172 := FALSE;
   Allar_173 := FALSE;
   Allar_174 := FALSE;
   Allar_175 := TRUE;
   Allar_176 := FALSE;
   Allar_161 := FALSE;
   Allar_162 := FALSE;
   Allar_163 := FALSE;
   Allar_164 := FALSE;
   Allar_165 := FALSE;
   Allar_166 := FALSE;
   Allar_167 := FALSE;
   Allar_168 := FALSE;
   Allar_185 := FALSE;
   Allar_186 := FALSE;
   Allar_187 := FALSE;
   Allar_188 := FALSE;
   Allar_189 := FALSE;
   Allar_190 := FALSE;
   Allar_191 := FALSE;
   Allar_192 := FALSE;
   Allar_177 := FALSE;
   Allar_178 := FALSE;
   Allar_179 := FALSE;
   Allar_180 := FALSE;
   Allar_181 := FALSE;
   Allar_182 := FALSE;
   Allar_183 := FALSE;
   Allar_184 := FALSE;
   word_3042 := FALSE;
   word_3043 := FALSE;
   word_3044 := FALSE;
   word_3045 := FALSE;
   word_3046 := FALSE;
   word_3047 := FALSE;
   word_3048 := FALSE;
   word_3049 := FALSE;
   word_3050 := FALSE;
   word_3051 := FALSE;
   word_3052 := FALSE;
   word_3053 := FALSE;
   word_3054 := FALSE;
   word_3055 := FALSE;
   word_3056 := FALSE;
   word_3057 := FALSE;
   Allar_217 := FALSE;
   Allar_218 := FALSE;
   Allar_219 := FALSE;
   Allar_220 := FALSE;
   Allar_221 := FALSE;
   word_3063 := FALSE;
   word_3064 := FALSE;
   word_3065 := FALSE;
   Allar_209 := FALSE;
   Allar_210 := FALSE;
   Allar_211 := FALSE;
   Allar_212 := FALSE;
   Allar_213 := FALSE;
   word_30635 := FALSE;
   word_30636 := FALSE;
   word_30637 := FALSE;
   word_30638 := FALSE;
   word_30639 := FALSE;
   word_306310 := FALSE;
   word_306311 := FALSE;
   word_306312 := FALSE;
   word_306313 := FALSE;
   word_306314 := FALSE;
   word_306315 := FALSE;
   Allar_225 := FALSE;
   word_3063152 := FALSE;
   word_3063153 := FALSE;
   word_30631531 := FALSE;
   word_30631532 := FALSE;
   word_30631533 := FALSE;
   word_30631534 := FALSE;
   word_30631535 := FALSE;
   Da_APT_allarme_1 := FALSE;
   Da_APT_allarme_2 := FALSE;
   Da_APT_allarme_3 := FALSE;
   Da_APT_allarme_4 := FALSE;
   Da_APT_allarme_5 := FALSE;
   Da_APT_allarme_6 := FALSE;
   Da_APT_allarme_7 := FALSE;
   Da_APT_allarme_8 := FALSE;
   Da_APT_allarme_9 := FALSE;
   Da_APT_allarme_10 := FALSE;
   Da_APT_allarme_11 := FALSE;
   Da_APT_allarme_12 := FALSE;
   Da_APT_allarme_13 := FALSE;
   Da_APT_allarme_14 := FALSE;
   Da_APT_allarme_15 := FALSE;
   Da_APT_allarme_16 := FALSE;
   Da_APT_allarme_17 := FALSE;
   Da_APT_allarme_18 := FALSE;
   Da_APT_allarme_19 := FALSE;
   Da_APT_allarme_20 := FALSE;
   Da_APT_allarme_21 := FALSE;
   Da_APT_allarme_22 := FALSE;
   Da_APT_allarme_23 := FALSE;
   Da_APT_allarme_24 := FALSE;
   Da_APT_allarme_25 := FALSE;
   Da_APT_allarme_26 := FALSE;
   Da_APT_allarme_27 := FALSE;
   Da_APT_allarme_28 := FALSE;
   Da_APT_allarme_29 := FALSE;
   Da_APT_allarme_30 := FALSE;
   Da_APT_allarme_31 := FALSE;
   Da_APT_allarme_32 := FALSE;
   Da_APT_allarme_33 := FALSE;
   Da_APT_allarme_34 := FALSE;
   Da_APT_allarme_35 := FALSE;
   Da_APT_allarme_36 := FALSE;
   Da_APT_allarme_37 := FALSE;
   Da_APT_allarme_38 := FALSE;
   Da_APT_allarme_39 := FALSE;
   Da_APT_allarme_40 := FALSE;
   Da_APT_allarme_41 := FALSE;
   Da_APT_allarme_42 := FALSE;
   Da_APT_allarme_43 := FALSE;
   Da_APT_allarme_44 := FALSE;
   Da_APT_allarme_45 := FALSE;
   Da_APT_allarme_46 := FALSE;
   Da_APT_allarme_47 := FALSE;
   Da_APT_allarme_48 := FALSE;
   Da_APT_allarme_49 := FALSE;
   Da_APT_allarme_50 := FALSE;
   Da_APT_allarme_51 := FALSE;
   Da_APT_allarme_52 := FALSE;
   Da_APT_allarme_53 := FALSE;
   Da_APT_allarme_54 := FALSE;
   Da_APT_allarme_55 := FALSE;
   Da_APT_allarme_56 := FALSE;
   Da_APT_allarme_57 := FALSE;
   Da_APT_allarme_58 := FALSE;
   Da_APT_allarme_59 := FALSE;
   Da_APT_allarme_60 := FALSE;
   Da_APT_allarme_61 := FALSE;
   Da_APT_allarme_62 := FALSE;
   Da_APT_allarme_63 := FALSE;
   Da_APT_allarme_64 := FALSE;
   Da_APT_allarme_65 := FALSE;
   Da_APT_allarme_66 := FALSE;
   Da_APT_allarme_67 := FALSE;
   Da_APT_allarme_68 := FALSE;
   Da_APT_allarme_69 := FALSE;
   Da_APT_allarme_70 := FALSE;
   Da_APT_allarme_71 := FALSE;
   Da_APT_allarme_72 := FALSE;
   Da_APT_allarme_73 := FALSE;
   Da_APT_allarme_74 := FALSE;
   Da_APT_allarme_75 := FALSE;
   Da_APT_allarme_76 := FALSE;
   Da_APT_allarme_77 := FALSE;
   Da_APT_allarme_78 := FALSE;
   Da_APT_allarme_79 := FALSE;
   Da_APT_allarme_80 := FALSE;
   Da_APT_allarme_81 := FALSE;
   Da_APT_allarme_82 := FALSE;
   Da_APT_allarme_83 := FALSE;
   Da_APT_allarme_84 := FALSE;
   Da_APT_allarme_85 := FALSE;
   Da_APT_allarme_86 := FALSE;
   Da_APT_allarme_87 := FALSE;
   Da_APT_allarme_88 := FALSE;
   Da_APT_allarme_89 := FALSE;
   Da_APT_allarme_90 := FALSE;
   Da_APT_allarme_91 := FALSE;
   Da_APT_allarme_92 := FALSE;
   Da_APT_allarme_93 := FALSE;
   Da_APT_allarme_94 := FALSE;
   Da_APT_allarme_95 := FALSE;
   Da_APT_allarme_96 := FALSE;
   Da_APT_allarme_97 := FALSE;
   Da_APT_allarme_98 := FALSE;
   Da_APT_allarme_99 := FALSE;
   Da_APT_allarme_100 := FALSE;
   Da_APT_allarme_101 := FALSE;
   Da_APT_allarme_102 := FALSE;
   Da_APT_allarme_103 := FALSE;
   Da_APT_allarme_104 := FALSE;
   Da_APT_allarme_105 := FALSE;
   Da_APT_allarme_106 := FALSE;
   Da_APT_allarme_107 := FALSE;
   Da_APT_allarme_108 := FALSE;
   Da_APT_allarme_109 := FALSE;
   Da_APT_allarme_110 := FALSE;
   Da_APT_allarme_111 := FALSE;
   Da_APT_allarme_112 := FALSE;
   Da_APT_allarme_113 := FALSE;
   Da_APT_allarme_114 := FALSE;
   Da_APT_allarme_115 := FALSE;
   Da_APT_allarme_116 := FALSE;
   Da_APT_allarme_117 := FALSE;
   Da_APT_allarme_118 := FALSE;
   Da_APT_allarme_119 := FALSE;
   Da_APT_allarme_120 := FALSE;
   Da_APT_allarme_121 := FALSE;
   Da_APT_allarme_122 := FALSE;
   Da_APT_allarme_123 := FALSE;
   Da_APT_allarme_124 := FALSE;
   Da_APT_allarme_125 := FALSE;
   Da_APT_allarme_126 := FALSE;
   Da_APT_allarme_127 := FALSE;
   Da_APT_allarme_128 := FALSE;
   Da_APT_allarme_129 := FALSE;
   Da_APT_allarme_130 := FALSE;
   Da_APT_allarme_131 := FALSE;
   Da_APT_allarme_132 := FALSE;
   Da_APT_allarme_133 := FALSE;
   Da_APT_allarme_134 := FALSE;
   Da_APT_allarme_135 := FALSE;
   Da_APT_allarme_136 := FALSE;
   Da_APT_allarme_137 := FALSE;
   Da_APT_allarme_138 := FALSE;
   Da_APT_allarme_139 := FALSE;
   Da_APT_allarme_140 := FALSE;
   Da_APT_allarme_141 := FALSE;
   Da_APT_allarme_142 := FALSE;
   Da_APT_allarme_143 := FALSE;
   Da_APT_allarme_144 := FALSE;
   Da_APT_allarme_145 := FALSE;
   Da_APT_allarme_146 := FALSE;
   Da_APT_allarme_147 := FALSE;
   Da_APT_allarme_148 := FALSE;
   Da_APT_allarme_149 := FALSE;
   Da_APT_allarme_150 := FALSE;
   Da_APT_allarme_151 := FALSE;
   Da_APT_allarme_152 := FALSE;
   Da_APT_allarme_153 := FALSE;
   Da_APT_allarme_154 := FALSE;
   Da_APT_allarme_155 := FALSE;
   Da_APT_allarme_156 := FALSE;
   Da_APT_allarme_157 := FALSE;
   Da_APT_allarme_158 := FALSE;
   Da_APT_allarme_159 := FALSE;
   Da_APT_allarme_160 := FALSE;
END_DATA_BLOCK

